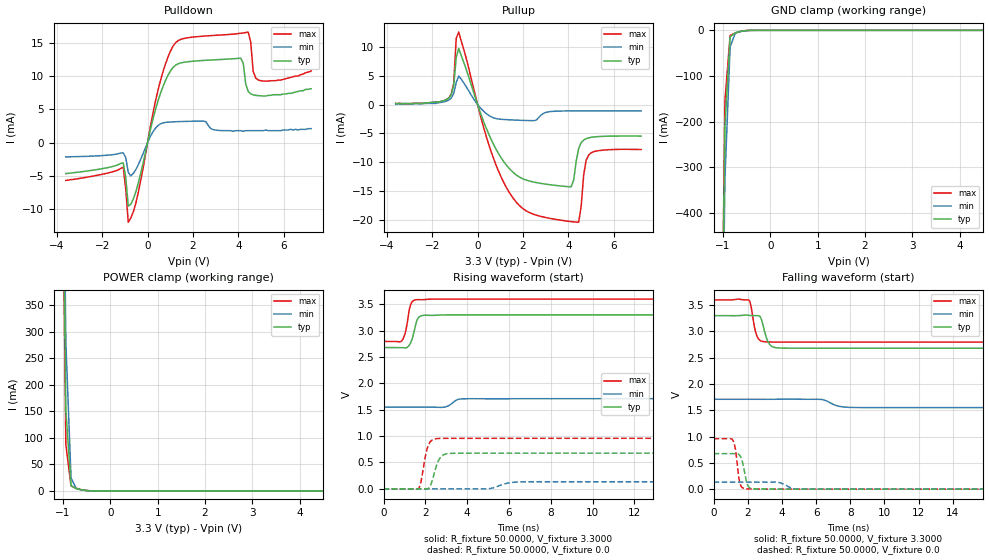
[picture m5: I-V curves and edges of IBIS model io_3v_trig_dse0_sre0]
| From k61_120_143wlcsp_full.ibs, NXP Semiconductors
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[Model]  io_3v_trig_dse0_sre0
|   Model io_3v_trig_dse0_sre0
| Library cells for typ/min/max conditions are connected as defined below:
|  pad - External Pad
|  ipp_do_3v - Core Input
|  ipp_obe_3v - Output Buffer Enable
|  esd_boost - vdd_s_3v
|  esd_trigger - vss_s_3v
|  ipp_ame_3v - vss_s_3v
|  ipp_dse_3v - vss_s_3v
|  ipp_ina_3v - NC
|  ipp_ina_mux_3v - NC
|  ipp_ind_3v - NC
|  ipp_pue_3v - vss_s_3v
|  ipp_sre_3v - vss_s_3v
|  tie_3v - vdd_s_3v
|  tie_hi - vdd_s_lv
|  vbuf_3v - vdd_s_3v
|  vdd_s_3v - vdd_s_3v
|  vdd_s_lv - vdd_s_lv
|  vss_bulk - vss_s_3v
|  vss_s_3v - vss_s_3v
| All other pins connected to ground
Model_type I/O
Polarity   Non-Inverting
Enable   Active-High
Vinl =   1.1550V
Vinh =   2.3100V
Vmeas =  1.6500V
Cref =   25.0000pF
Rref =   50.0000
Vref =   0.0V
C_comp   1.9033pF   1.7921pF   2.1182pF
[Temperature Range]   25.0000   0.1250k   -40.0000
[Voltage Range]   3.3000V   1.7100V   3.6000V
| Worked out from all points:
|   slope of the pulldown table from 0 to 0.495 V, typ, clamps not added: 74.6 ohm
|   slope of the pullup table from 0 to 0.495 V, typ, clamps not added: 96.1 ohm
|   GND clamp passes 1 mA (typ) near -0.54 V on its own axis
|   POWER clamp passes 1 mA (typ) near -0.53 V on its own axis
|   rising waveform, R_fixture 50.0000, V_fixture 3.3000: 20-80 % time 249ps typ, 324ps min, 218ps max; typ from 2.68 V to 3.3 V
|   rising waveform, R_fixture 50.0000, V_fixture 0.0: 20-80 % time 324ps typ, 610ps min, 273ps max; typ from 0 V to 0.676 V
|   falling waveform, R_fixture 50.0000, V_fixture 3.3000: 20-80 % time 336ps typ, 646ps min, 278ps max; typ from 3.3 V to 2.68 V
|   falling waveform, R_fixture 50.0000, V_fixture 0.0: 20-80 % time 264ps typ, 480ps min, 219ps max; typ from 0.676 V to 0 V
[Pulldown]
|Voltage   I(typ)   I(min)   I(max)
-3.6V     -4.64mA    -2.13mA    -5.68mA
-1.07V    -3.05mA    -1.536mA   -3.686mA
-850mV    -9.531mA   -4.459mA   -11.94mA
-520mV    -7.433mA   -4.073mA   -9.157mA
580mV     7.512mA    2.843mA    9.473mA
1.46V     11.97mA    3.168mA    15.51mA
4.1V      12.68mA    1.8mA      16.42mA
4.43V     7.69mA     1.8mA      16.6mA
4.54V     7.33mA     1.8mA      15.1mA
4.65V     7.17mA     1.8mA      10.69mA
4.87V     7.06mA     1.8mA      9.41mA
7.2V      8.1mA      2.1mA      10.8mA
[Pullup]
|Voltage   I(typ)   I(min)   I(max)
-3.6V     200uA      0A         200uA
-1.27V    1.12mA     760uA      1.13mA
-1.05V    3.27mA     1.9mA      3.696mA
-940mV    8.16mA     3.801mA    11.47mA
-830mV    9.694mA    4.923mA    12.52mA
1.15V     -9.866mA   -2.586mA   -13.47mA
3.24V     -13.9mA    -1.205mA   -19.73mA
4.12V     -14.22mA   -1.1mA     -20.25mA
4.45V     -7.608mA   -1.09mA    -20.35mA
4.78V     -5.902mA   -1.09mA    -9.632mA
5V        -5.67mA    -1.1mA     -8.343mA
7.2V      -5.46mA    -1.11mA    -7.78mA
[GND_clamp]
|Voltage   I(typ)   I(min)   I(max)
-3.6V     -47.82A    -47.1A     -48.34A
-1.07V    -1.102A    -1.183A    -1.105A
-960mV    -210.7mA   -326mA     -154mA
-850mV    -14.47mA   -36.11mA   -11.11mA
-740mV    -5.262mA   -6.033mA   -5.843mA
-520mV    -636.9uA   -915.4uA   -467.5uA
-300mV    -2.578uA   -18.09uA   -370.9nA
7.2V      0A         0A         0A
[POWER_clamp]
|Voltage   I(typ)   I(min)   I(max)
-3.6V     36.98A     36.74A     37.19A
-1.05V    1.02A      1.161A     949.9mA
-940mV    152.3mA    280.6mA    87.35mA
-830mV    9.987mA    24.48mA    9.181mA
-720mV    4.227mA    4.408mA    5.116mA
-500mV    628.6uA    743.9uA    622.6uA
-390mV    66.57uA    164uA      29.9uA
7.2V      0A         0A         0A
[Ramp]
| variable   typ   min   max
dV/dt_r  0.4057/0.3234n   80.2999m/0.6106n   0.5756/0.2727n
dV/dt_f  0.3715/0.3360n   95.2938m/0.6465n   0.4821/0.2780n
R_load = 50.0000
[Rising Waveform]
R_fixture= 50.0000
V_fixture= 3.3000
V_fixture_min= 1.7100
V_fixture_max= 3.6000
|time   V(typ)   V(min)   V(max)
0s        2.681V     1.551V     2.796V
881.7ps   2.678V     1.551V     2.812V
1.026ns   2.672V     1.551V     2.94V
1.299ns   2.77V      1.552V     3.498V
1.593ns   3.192V     1.552V     3.59V
1.844ns   3.287V     1.551V     3.588V
2.927ns   3.299V     1.55V      3.6V
3.555ns   3.3V       1.695V     3.6V
3.921ns   3.3V       1.709V     3.6V
20ns      3.3V       1.71V      3.6V
[Rising Waveform]
R_fixture= 50.0000
V_fixture= 0.0
V_fixture_min= 0.0
V_fixture_max= 0.0
|time   V(typ)   V(min)   V(max)
0s        5.332nV    455.6nV    4.027nV
1.688ns   -2.656mV   8.137uV    13.65mV
1.793ns   -1.209mV   11.32uV    135.1mV
2.13ns    5.672mV    34.21uV    818.1mV
2.293ns   111.3mV    45.93uV    915.7mV
2.511ns   412.6mV    41.14uV    950.9mV
2.86ns    644.5mV    -155.2uV   957.7mV
3.311ns   674.1mV    -1.413mV   958.6mV
6.757ns   675.9mV    132.6mV    959mV
20ns      676.2mV    133.8mV    959.4mV
[Falling Waveform]
R_fixture= 50.0000
V_fixture= 3.3000
V_fixture_min= 1.7100
V_fixture_max= 3.6000
|time   V(typ)   V(min)   V(max)
0s        3.3V       1.71V      3.6V
2.059ns   3.307V     1.71V      3.599V
2.542ns   3.3V       1.71V      2.907V
2.728ns   3.282V     1.71V      2.829V
3.008ns   2.971V     1.71V      2.803V
3.282ns   2.752V     1.71V      2.8V
3.912ns   2.685V     1.711V     2.798V
6.337ns   2.681V     1.707V     2.797V
7.895ns   2.681V     1.557V     2.797V
20ns      2.681V     1.551V     2.796V
[Falling Waveform]
R_fixture= 50.0000
V_fixture= 0.0
V_fixture_min= 0.0
V_fixture_max= 0.0
|time   V(typ)   V(min)   V(max)
0s        676.3mV    133.9mV    959.6mV
1.138ns   677.2mV    133.9mV    928.2mV
1.283ns   677.9mV    133.8mV    754.8mV
1.523ns   647.2mV    133.8mV    138.4mV
1.698ns   511.3mV    133.8mV    25.35mV
1.847ns   266.1mV    133.8mV    7.41mV
2.05ns    43.85mV    133.8mV    4.19mV
2.372ns   3.527mV    133.9mV    3.217mV
4.936ns   257.9uV    1.307mV    352.6uV
20ns      97.17uV    25.98uV    132.2uV
